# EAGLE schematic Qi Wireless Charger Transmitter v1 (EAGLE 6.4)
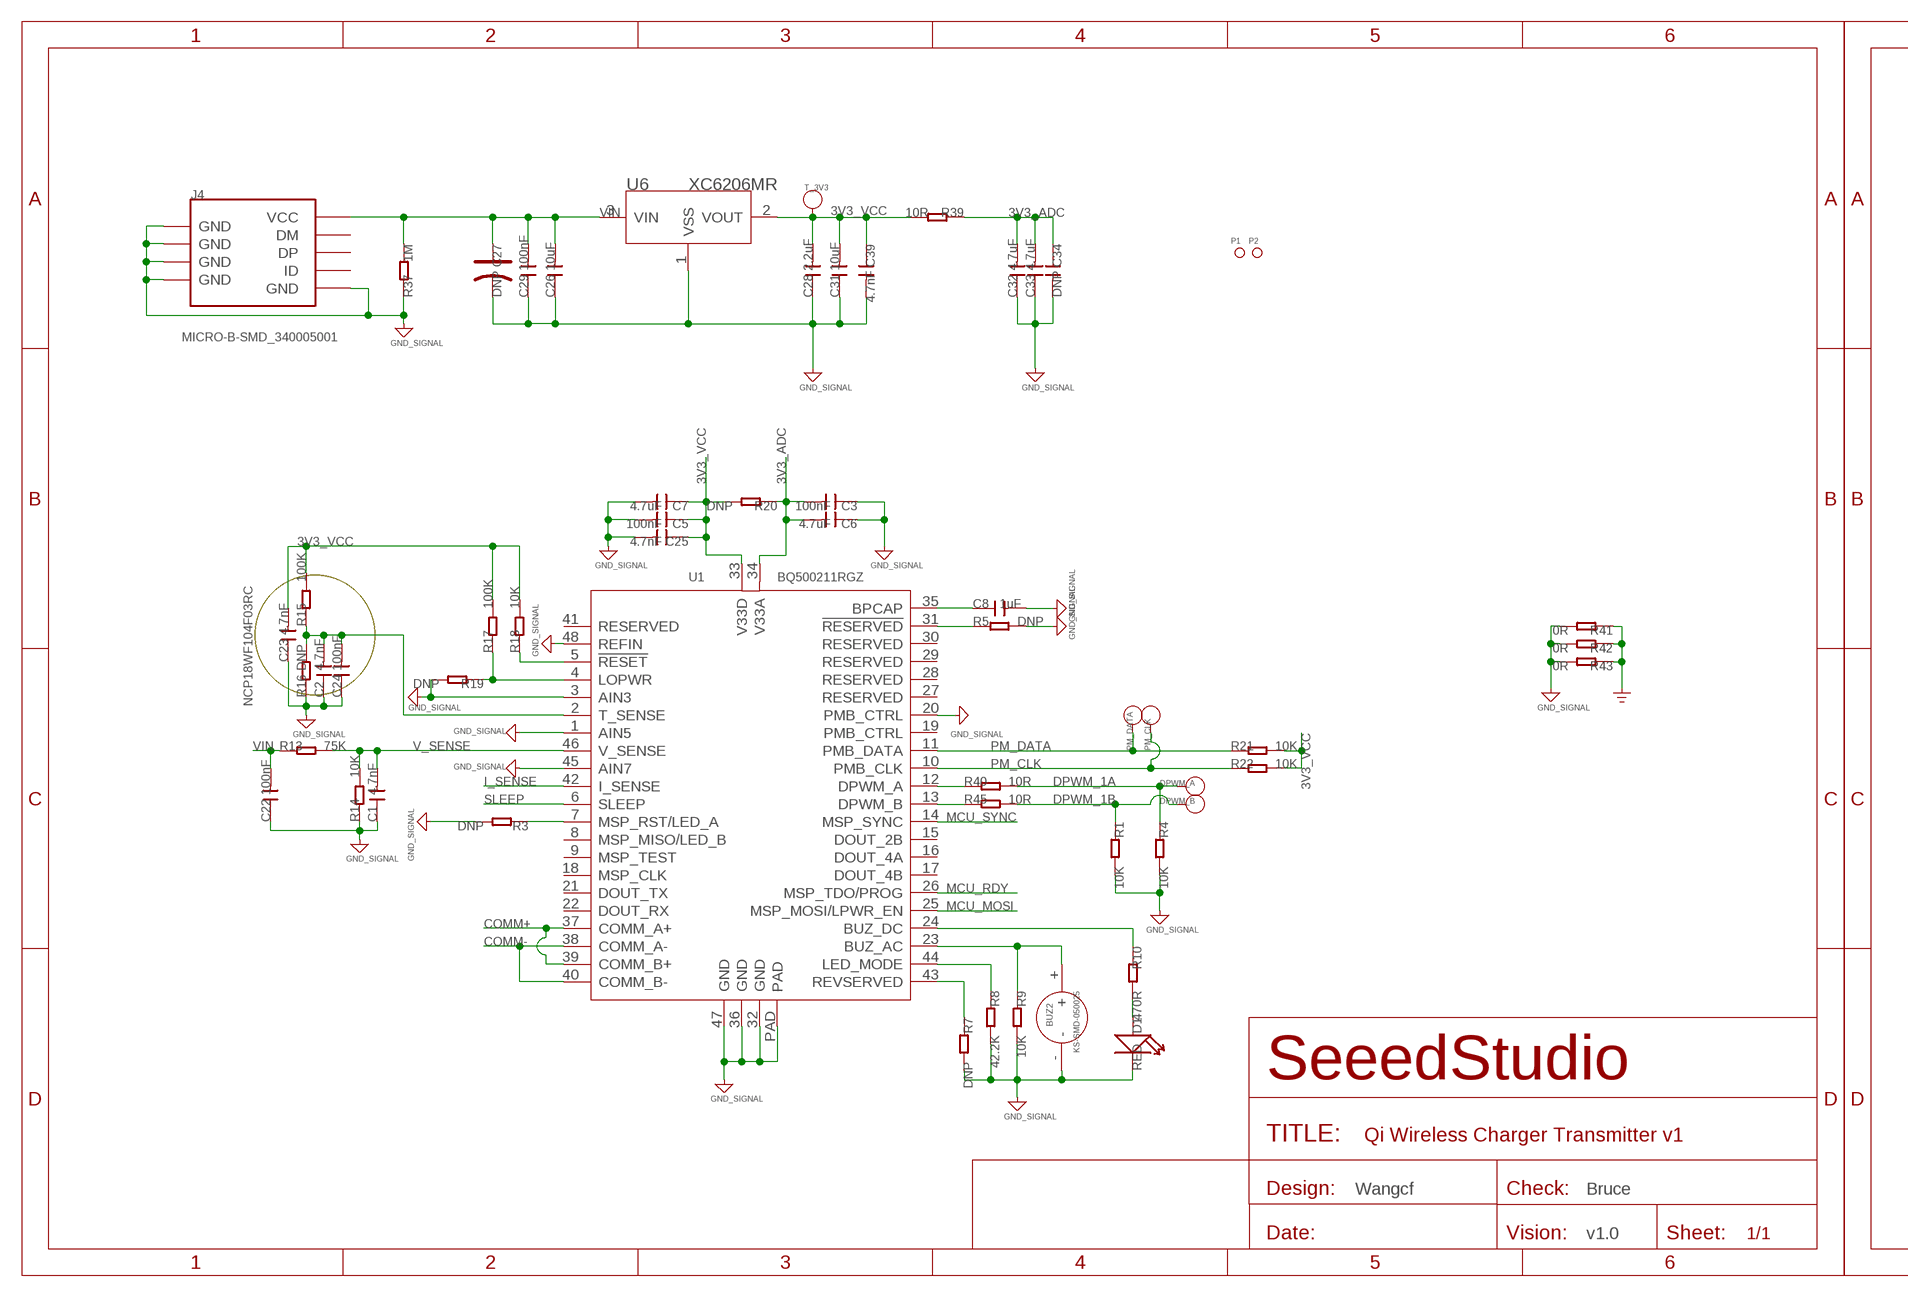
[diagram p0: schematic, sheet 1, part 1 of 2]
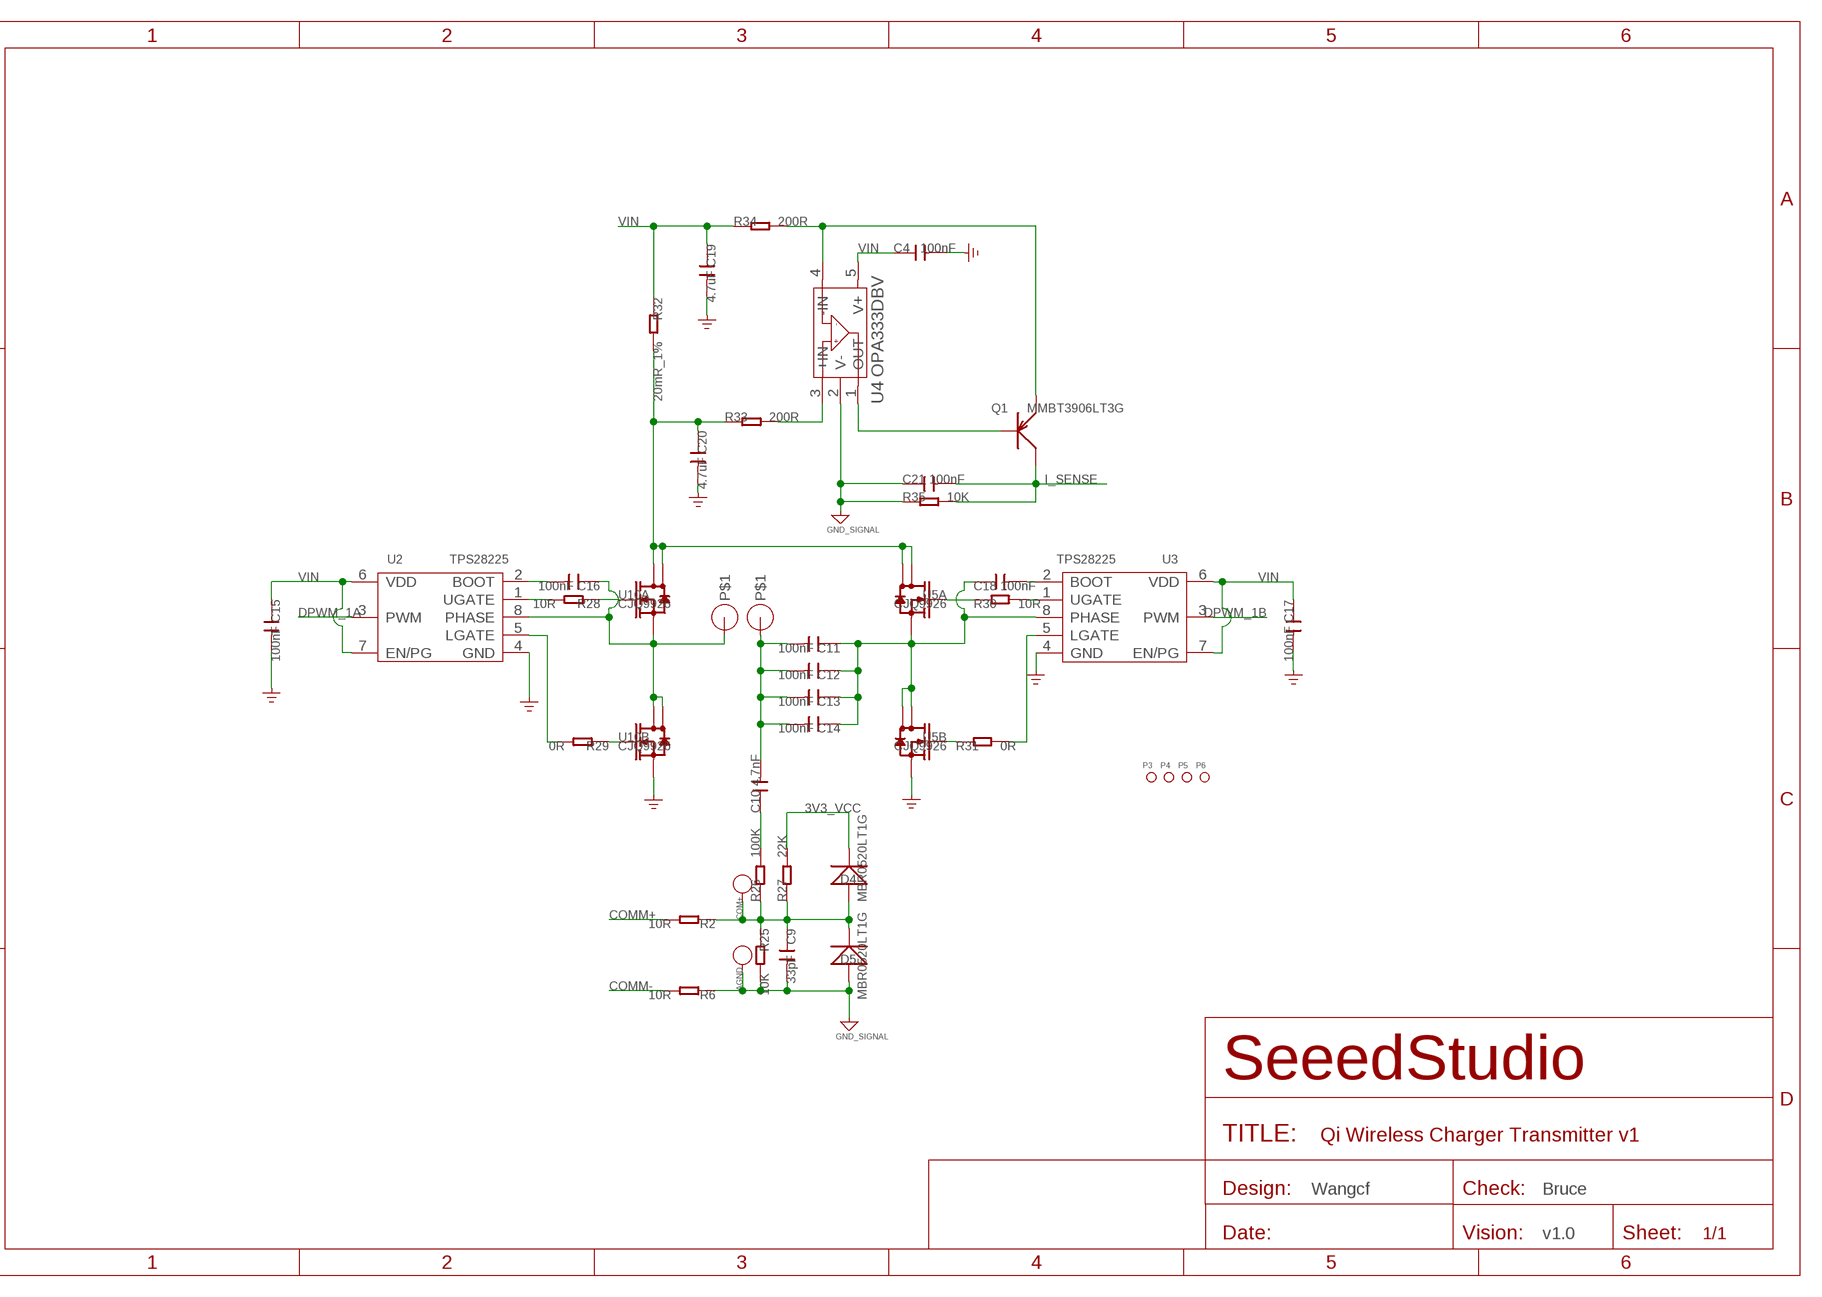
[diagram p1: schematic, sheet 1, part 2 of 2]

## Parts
AGND  DNP  PAD-TEST-POINT'4545'  [TP_4545]
BUZ2  KS-SMD-050025  BUZZER'KS-SMD-050025'  [3P-5X5X2.5H]
C1  4.7nF  C-0603  [C0603]
C2  4.7nF  C-0603  [C0603]
C3  100nF  C-0603  [C0603]
C4  100nF  C-0603  [C0603]
C5  100nF  C-0603  [C0603]
C6  4.7uF  C-0805  [C0805]
C7  4.7uF  C-0805  [C0805]
C8  1uF  C-0603  [C0603]
C9  33pF  C-0603  [C0603]
C10  4.7nF  C-0603  [C0603]
C11  100nF  C-1206  [C1206]
C12  100nF  C-1206  [C1206]
C13  100nF  C-1206  [C1206]
C14  100nF  C-1206  [C1206]
C15  100nF  C-0603  [C0603]
C16  100nF  C-0603  [C0603]
C17  100nF  C-0603  [C0603]
C18  100nF  C-0603  [C0603]
C19  4.7uF  C-0805  [C0805]
C20  4.7uF  C-0805  [C0805]
C21  100nF  C-0603  [C0603]
C22  100nF  C-0603  [C0603]
C23  4.7nF  C-0603  [C0603]
C24  100nF  C-0603  [C0603]
C25  4.7nF  C-0603  [C0603]
C26  10uF  C-0805  [C0805]
C27  DNP  CAP-AVX-B  [AVX-B]
C28  2.2uF  C-0805  [C0805]
C29  100nF  C-0603  [C0603]
C31  10uF  C-0805  [C0805]
C32  4.7uF  C-0805  [C0805]
C33  4.7uF  C-0805  [C0805]
C34  DNP  C-0603  [C0603]
C39  4.7nF  C-0603  [C0603]
COII2  PAD-HOLE  [1P-220X140]
COIL1  PAD-HOLE  [1P-220X140]
COM+  DNP  PAD-TEST-POINT'4545'  [TP_4545]
D1  RED  LED'0603'  [LED-0603]
D4  MBR0520LT1G  D-SOD-123  [SOD123]
D5  MBR0520LT1G  D-SOD-123  [SOD123]
DPWM_A  DNP  PAD-TEST-POINT'4545'  [TP_4545]
DPWM_B  DNP  PAD-TEST-POINT'4545'  [TP_4545]
J4  MICRO-B-SMD_340005001  USB-MINIUSB-5P-MICRO  [MICRO-USB]
P1  PAD-MARK'ANNULAR'  [ROUND-MARK-1.0]
P2  PAD-MARK'ANNULAR'  [ROUND-MARK-1.0]
P3  PAD-MARK'ANNULAR'  [ROUND-MARK-1.0]
P4  PAD-MARK'ANNULAR'  [ROUND-MARK-1.0]
P5  PAD-MARK'ANNULAR'  [ROUND-MARK-1.0]
P6  PAD-MARK'ANNULAR'  [ROUND-MARK-1.0]
PM_CLK  DNP  PAD-TEST-POINT'4545'  [TP_4545]
PM_DATA  DNP  PAD-TEST-POINT'4545'  [TP_4545]
Q1  MMBT3906LT3G  TRANSISTOR-PNP-SOT23  [SOT23]
R1  10K  R-0603  [R0603]
R2  10R  R-0603  [R0603]
R3  DNP  R-0603  [R0603]
R4  10K  R-0603  [R0603]
R5  DNP  R-0603  [R0603]
R6  10R  R-0603  [R0603]
R7  DNP  R-0603  [R0603]
R8  42.2K  R-0603  [R0603]
R9  10K  R-0603  [R0603]
R10  470R  R-0603  [R0603]
R13  75K  R-0603  [R0603]
R14  10K  R-0603  [R0603]
R15  100K  R-0603  [R0603]
R16  DNP  R-0603  [R0603]
R17  100K  R-0603  [R0603]
R18  10K  R-0603  [R0603]
R19  DNP  R-0603  [R0603]
R20  DNP  R-0603  [R0603]
R21  10K  R-0603  [R0603]
R22  10K  R-0603  [R0603]
R25  10K  R-0603  [R0603]
R26  100K  R-0603  [R0603]
R27  22K  R-0603  [R0603]
R28  10R  R-0603  [R0603]
R29  0R  R-0603  [R0603]
R30  10R  R-0603  [R0603]
R31  0R  R-0603  [R0603]
R32  20mR_1%  R-2512  [R2512]
R33  200R  R-0603  [R0603]
R34  200R  R-0603  [R0603]
R35  10K  R-0603  [R0603]
R37  1M  R-0603  [R0603]
R39  10R  R-0603  [R0603]
R40  10R  R-0603  [R0603]
R41  0R  R-0603  [R0603]
R42  0R  R-0603  [R0603]
R43  0R  R-0603  [R0603]
R45  10R  R-0603  [R0603]
T_3V3  DNP  PAD-TEST-POINT-CIRCLE'4545'  [TP_4545]
U1  BQ500211RGZ  BQ500211'RGZ'  [VQFN48]
U2  TPS28225  TPS28225'D'  [SOIC8-6.0]
U3  TPS28225  TPS28225'D'  [SOIC8-6.0]
U4  OPA333DBV  [SOT23-5]
U5  CJQ9926  MOSFET-DUAL-N-SOP08  [SOP8]
U6  XC6206MR  [SOT23]
U10  CJQ9926  MOSFET-DUAL-N-SOP08  [SOP8]

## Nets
3V3_ADC: C3.2 C6.2 C32.2 C33.2 C34.1 R20.1 R39.1 U1.34(V33A)
3V3_VCC: C5.1 C7.1 C23.2 C25.1 C28.2 C31.2 C39.1 D4.- R15.2 R17.2 R18.2 R20.2 R21.2 R22.2 R27.2 R39.2 T_3V3.T U1.33(V33D) U6.2(VOUT)
AGND: AGND.T BUZ2.- C1.1 C2.1 C3.1 C5.2 C6.1 C7.2 C8.2 C9.2 C21.1 C22.1 C23.1 C24.1 C25.2 C26.1 C27.- C28.1 C29.1 C31.1 C32.1 C33.1 C34.2 C39.2 D1.- D5.+ J4.5(GND) J4.S1(GND) J4.S2(GND) J4.S3(GND) J4.S4(GND) J4.S5(GND) J4.S6(GND) R1.2 R3.2 R4.2 R5.2 R6.1 R7.2 R8.2 R9.2 R14.1 R16.1 R19.2 R25.2 R35.1 R37.1 R41.2 R42.2 R43.2 U1.1(AIN5) U1.3(AIN3) U1.20(PMB_CTRL) U1.32(GND) U1.36(GND) U1.45(AIN7) U1.47(GND) U1.48(REFIN) U1.PAD U4.2(V-) U6.1(VSS) ; supply symbol labelled GND_SIGNAL
COMM+: R2.2 U1.37(COMM_A+) U1.39(COMM_B+)
COMM-: R6.2 U1.38(COMM_A-) U1.40(COMM_B-)
DPWM_1A: DPWM_A.T R4.1 R40.2 U2.3(PWM)
DPWM_1B: DPWM_B.T R1.1 R45.2 U3.3(PWM)
GND: C4.2 C15.2 C17.2 C19.2 C20.2 R41.1 R42.1 R43.1 U2.4(GND) U3.4(GND) U5.3(B:S) U10.3(B:S)
I_SENSE: C21.2 Q1.3(C) R35.2 U1.42(I_SENSE)
LOSS_THR: R7.1 U1.43(REVSERVED)
MCU_MOSI: U1.25(MSP_MOSI/LPWR_EN)
MCU_RDY: U1.26(MSP_TDO/PROG)
MCU_SYNC: U1.14(MSP_SYNC)
N$2: R5.1 U1.31(!RESERVED)
N$3: R3.1 U1.7(MSP_RST/LED_A)
N$5: R45.1 U1.13(DPWM_B)
N$6: R40.1 U1.12(DPWM_A)
N$7: C9.1 COM+.T D4.+ D5.- R2.1 R25.1 R26.1 R27.1
N$8: R33.2 U4.3(+IN)
N$10: C2.2 C24.2 R15.1 R16.2 U1.2(T_SENSE)
N$11: C10.1 R26.2
N$12: R8.1 U1.44(LED_MODE)
N$13: BUZ2.+ R9.1 U1.23(BUZ_AC)
N$14: D1.+ R10.2
N$15: R10.1 U1.24(BUZ_DC)
N$17: C8.1 U1.35(BPCAP)
N$18: R29.2 U2.5(LGATE)
N$19: R18.1 U1.5(!RESET)
N$20: R17.1 R19.1 U1.4(LOPWR)
N$21: R28.2 U2.1(UGATE)
N$22: C18.2 U3.2(BOOT)
N$24: C16.1 COII2.P$1 U2.8(PHASE) U10.1(A:S) U10.5(B:D) U10.6(B:D)
N$25: R28.1 U10.2(A:G)
N$27: Q1.2(E) R34.2 U4.4(-IN)
N$28: R29.1 U10.4(B:G)
N$29: C16.2 U2.2(BOOT)
N$30: R31.2 U3.5(LGATE)
N$31: R30.1 U5.2(A:G)
N$33: R31.1 U5.4(B:G)
N$34: R30.2 U3.1(UGATE)
N$35: C11.1 C12.1 C13.1 C14.1 C18.1 U3.8(PHASE) U5.1(A:S) U5.5(B:D) U5.6(B:D)
N$37: C10.2 C11.2 C12.2 C13.2 C14.2 COIL1.P$1
N$40: C20.1 R32.2 R33.1 U5.7(A:D) U5.8(A:D) U10.7(A:D) U10.8(A:D)
N$41: Q1.1(B) U4.1(OUT)
PM_CLK: PM_CLK.T R22.1 U1.10(PMB_CLK)
PM_DATA: PM_DATA.T R21.1 U1.11(PMB_DATA)
SLEEP: U1.6(SLEEP)
V_SENSE: C1.2 R13.2 R14.2 U1.46(V_SENSE)
VIN: C4.1 C15.1 C17.1 C19.1 C22.2 C26.2 C27.+ C29.2 J4.1(VCC) R13.1 R32.1 R34.1 R37.2 U2.6(VDD) U2.7(EN/PG) U3.6(VDD) U3.7(EN/PG) U4.5(V+) U6.3(VIN)
Unconnected: J4.2(DM) J4.3(DP) J4.4(ID) U1.8(MSP_MISO/LED_B) U1.9(MSP_TEST) U1.15(DOUT_2B) U1.16(DOUT_4A) U1.17(DOUT_4B) U1.18(MSP_CLK) U1.19(PMB_CTRL) U1.21(DOUT_TX) U1.22(DOUT_RX) U1.27(RESERVED) U1.28(RESERVED) U1.29(RESERVED) U1.30(RESERVED) U1.41(RESERVED)

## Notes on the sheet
- NCP18WF104F03RC
- Wangcf | Bruce | Wangcf | Bruce
- v1.0 | v1.0

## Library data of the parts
AGND COM+ DPWM_A DPWM_B PM_CLK PM_DATA = Discrete:PAD-TEST-POINT; PARTNO: DNP
BUZ2 = template:BUZZER
C1-C26 C28 C29 C31-C34 C39 = Discrete:C*: Ceramic Capacitors
C27 = Discrete:CAP*: Electrolytic Capacitors,Tantalum Capacitors and Super Capacitors
COII2 COIL1 = Discrete:PAD-HOLE
D1 = Discrete:LED*
D4 D5 = OPL:D*: DIODE
J4 = Connector :USB-MINIUSB-5P
P1-P6 = Discrete:PAD-MARK; PARTNO: DNP
Q1 = Discrete:TRANSISTOR-PNP*: PNP audion
R1-R10 R13-R22 R25-R35 R37 R39-R43 R45 = Discrete:R*
T_3V3 = Discrete:PAD-TEST-POINT-CIRCLE; PARTNO: DNP
U1 = template:BQ500211
U2 U3 = template:TPS28225: High-Frequency 4-A Sink Synchronous MOSFET Drivers
U4 = IC:OPA333: 1.8V,Micro power CMOS oprational amplifiers Zero-Drift Series http://www.ti.com.cn/cn/lit/ds/symlink/opa333.pdf
U5 U10 = Discrete:MOSFET-DUAL-N: Si5902BDC/Si5904DC/Si5908DC/Si5920DC
U6 = IC:XC6206: LOW ESR Cap.Compatible Positive Voltage Regulators

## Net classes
0 default: width 0.003 mm, drill 0.254 mm, clearance 0.152 mm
